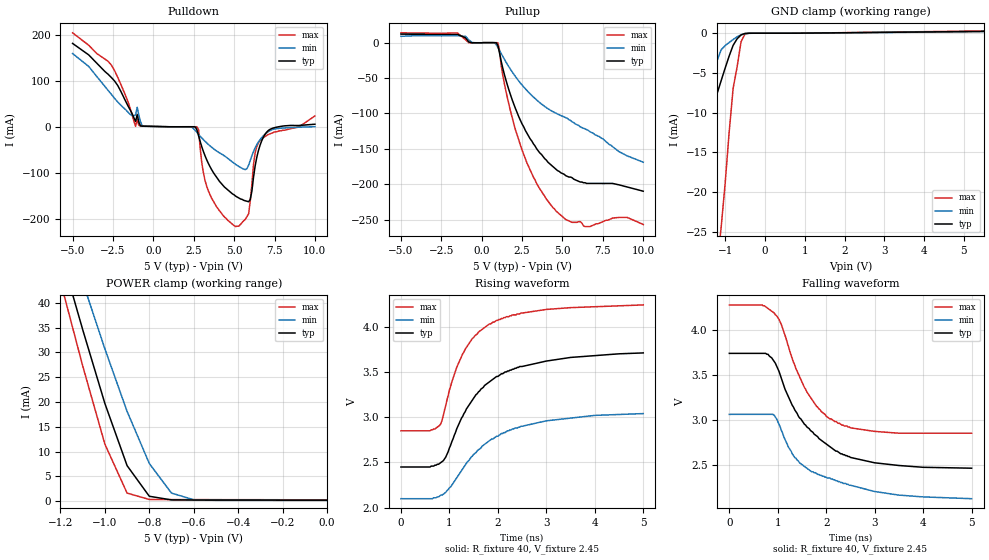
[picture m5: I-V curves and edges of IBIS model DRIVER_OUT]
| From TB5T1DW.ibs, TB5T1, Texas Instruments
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|   Driver Output Model
[Model]   DRIVER_OUT
Model_type   Output_ECL
| Signals   DO1,DO1(-),DO2,DO2(-)
Vmeas = 3.2V   |Reference voltage for timing measurements
Cref = 0pF   |Timing specification test load capacitance value
Rref = 40   |Note: 40 Ohm load; single ended configuration
| variable   typ   min   max
C_comp   970fF   930fF   1010fF
|   typ   min   max
[Temperature Range]   25.0   -40.0   125.0
[Voltage range]   5.0V   4.5V   5.5V
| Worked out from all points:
|   GND clamp passes 1 mA (typ) near -0.74 V on its own axis
|   POWER clamp passes 1 mA (typ) near -0.80 V on its own axis
|   rising waveform, R_fixture 40, V_fixture 2.45: 20-80 % time 987ps typ, 1.13ns min, 731ps max; typ from 2.45 V to 3.71 V
|   falling waveform, R_fixture 40, V_fixture 2.45: 20-80 % time 975ps typ, 1.2ns min, 714ps max; typ from 3.74 V to 2.46 V
[Pulldown]
|Voltage I(typ)   I(min)   I(max)
-5V       181mA      159mA      204mA
-2.6V     107mA      70.3mA     134mA
-1.1V     11.5mA     25.3mA     830uA
2.7V      -7.28mA    -12.5mA    -119uA
3.4V      -79.3mA    -38.3mA    -139mA
5.1V      -151mA     -82mA      -217mA
5.9V      -163mA     -83.4mA    -189mA
6V        -158mA     -73.1mA    -161mA
6.3V      -85.6mA    -46.1mA    -57.3mA
6.6V      -40.9mA    -28.4mA    -30.2mA
7.3V      -4.43mA    -7.11mA    -14.4mA
10V       5.42mA     36.8uA     23.4mA
[Pullup]
|   Voltage   I(typ)   I(min)   I(max)
| Note that the[Pullup]voltage table is referenced to Vcc
| and is calculated using Vtable=Vcc - Vmeasured.
-5V       12.1mA     8.97mA     13.9mA
-1.5V     11.7mA     9.75mA     13.7mA
-1V       6.79mA     8.88mA     4.07mA
1V        -3.83mA    -6.8mA     -208uA
1.6V      -60.7mA    -31.1mA    -79mA
2.5V      -115mA     -60mA      -152mA
3.4V      -150mA     -81mA      -199mA
4.4V      -175mA     -97.4mA    -233mA
5.2V      -188mA     -106mA     -250mA
6.4V      -198mA     -122mA     -260mA
8.5V      -201mA     -154mA     -247mA
10V       -210mA     -169mA     -257mA
[GND_clamp]
|   Voltage   I(typ)   I(min)   I(max)
| Outputs in High Impedance (off)
-5.5V     -216mA     -169mA     -280mA
-1.6V     -38.7mA    -41.9mA    -110mA
-1.5V     -18.9mA    -29.8mA    -72.8mA
-1.4V     -11.8mA    -17.5mA    -44.1mA
-1.3V     -9.26mA    -7.94mA    -36.7mA
-1.2V     -7.56mA    -3.42mA    -29.3mA
-1.1V     -5.96mA    -2.07mA    -24.4mA
-800mV    -1.53mA    -797uA     -6.95mA
-600mV    -217uA     -186uA     -1.06mA
-500mV    -20.4uA    -56.3uA    -92.9uA
-400mV    -1.07uA    -12.6uA    -4.4uA
5.5V      232uA      201uA      288uA
[Power_clamp]
| Note that the[POWER_clamp]voltage table is referenced to Vcc
| and is calculated using Vtable=Vcc - Vmeasured.
|Voltage  I(typ)   I(min)   I(max)
-5V       327mA      316mA      338mA
-1.2V     50.2mA     58.1mA     44.3mA
-1.1V     34.6mA     44.2mA     27.3mA
-1V       19.7mA     30.7mA     11.5mA
-900mV    7.17mA     18.1mA     1.64mA
-800mV    998uA      7.61mA     351uA
-700mV    264uA      1.64mA     328uA
-600mV    237uA      296uA      322uA
0V        207uA      154uA      285uA
[Ramp]
|   typ   min   max
dV/dt_r   0.774/1069ps   0.577/1207ps   0.858/804ps
dV/dt_f   0.774/979ps   0.575/1271ps   0.859/707ps
R_load = 40ohm
[Rising Waveform]
R_fixture = 40
V_fixture = 2.45
V_fixture_min = 2.05
V_fixture_max = 2.85
C_fixture = 0
|   V(typ)  V(min)  V(max)
0s        2.45V      2.1V       2.85V
800ps     2.49V      2.13V      2.91V
925ps     2.56V      2.17V      3.13V
1.05ns    2.73V      2.25V      3.39V
1.275ns   3.01V      2.43V      3.7V
1.475ns   3.19V      2.57V      3.87V
1.825ns   3.39V      2.74V      4.03V
2.45ns    3.56V      2.89V      4.14V
3ns       3.62V      2.96V      4.19V
5ns       3.71V      3.04V      4.24V
[Falling Waveform]
R_fixture = 40
V_fixture = 2.45
V_fixture_min = 2.05
V_fixture_max = 2.85
C_fixture = 0
|   V(typ)  V(min)  V(max)
0s        3.74V      3.06V      4.28V
750ps     3.74V      3.06V      4.26V
925ps     3.65V      3.05V      4.19V
1.075ns   3.46V      2.88V      4.06V
1.225ns   3.25V      2.69V      3.81V
1.45ns    3.02V      2.52V      3.48V
1.8ns     2.82V      2.4V       3.15V
2.175ns   2.66V      2.33V      2.98V
3ns       2.52V      2.2V       2.87V
5ns       2.46V      2.12V      2.85V
